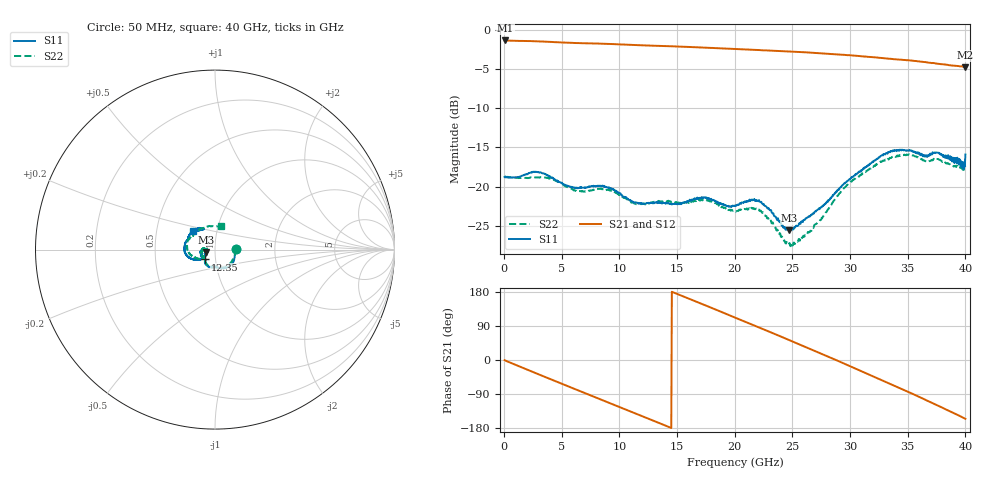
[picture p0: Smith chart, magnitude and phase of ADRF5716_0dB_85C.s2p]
! Device: ADRF5716
! Description: 30GHz 2-Bit Digital Attenuator
! Frequency: 100 MHz – 30 GHz
! Ports:
! ATTIN  = Port 1
! ATTOUT = Port 2
! State: 0 dB Attenuation selected
! Supply Voltage:
! VDD  =  +3.30 Volts
! VSS  =  -3.30 Volts
! Control Voltages:
! D5 = 0V, D6 = 0V
! Temperature = +85 C
! Data: Data was collected using a calibrated network analyzer.
!  The reference plane is the package pins of ADRF5716 switch.
! Note: Analog Devices supplies this data as a sample of measured data for this product.
!  Your particular data for this product may vary.
!  Analog Devices reserves the right to change this data at anytime
# HZ S DB R 50
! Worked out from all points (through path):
!   800 points, 50 MHz to 40 GHz, reference 50 ohm
!   highest |S21| = -1.40 dB at 100 MHz (marker M1); lowest = -4.8 dB at 40 GHz (marker M2)
!   group delay of S21, straight-line fit = 35.3 ps
!   lowest |S11| = -25.6 dB at 24.7 GHz (marker M3), VSWR 1.11, Z = 45.1 - j1.13 ohm
!   |S11| at or under -10 dB: start of sweep to end of sweep
!   |S22| runs from -27.6 to -15.9 dB; largest |S21 - S12| = 0
!   S11 on the Smith chart (normalised r, x): 50 MHz: 1.26, +0.01; 12.35 GHz: 0.89, -0.10; 40 GHz: 0.77, +0.16
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5e7  -18.79 1.2  -1.40 -0.6  -1.40 -0.6  -18.74 1.9
1e8  -18.76 -1.4  -1.40 -1.4  -1.40 -1.4  -18.73 -1.5
1.9e9  -18.45 -26.0  -1.46 -24.0  -1.46 -24.0  -18.89 -28.0
3.75e9  -18.53 -59.8  -1.56 -47.2  -1.56 -47.2  -18.92 -56.3
6.75e9  -20.13 -91.8  -1.74 -84.1  -1.74 -84.1  -20.65 -91.0
9.35e9  -20.31 -120.7  -1.85 -116.0  -1.85 -116.0  -20.55 -118.8
1.235e10  -22.12 -135.5  -2.03 -152.8  -2.03 -152.8  -22.13 -135.5
1.34e10  -22.05 -140.3  -2.08 -165.8  -2.08 -165.8  -21.83 -141.7
1.49e10  -22.23 -145.6  -2.16 175.7  -2.16 175.7  -21.98 -150.6
1.655e10  -21.57 -150.6  -2.25 155.4  -2.25 155.4  -21.84 -157.2
1.84e10  -21.87 -162.4  -2.37 132.5  -2.37 132.5  -22.13 -170.6
2.005e10  -22.39 -161.9  -2.48 111.6  -2.48 111.6  -23.08 -172.9
2.225e10  -22.01 -174.0  -2.64 84.0  -2.64 84.0  -23.06 176.6
2.47e10  -25.56 -166.3  -2.81 52.8  -2.81 52.8  -27.31 -173.8
2.67e10  -23.59 -150.1  -2.97 27.0  -2.97 27.0  -25.47 -149.2
2.83e10  -21.46 -145.0  -3.12 6.2  -3.12 6.2  -22.56 -143.9
2.99e10  -19.14 -148.4  -3.27 -14.9  -3.27 -14.9  -19.57 -150.9
3.335e10  -15.64 -172.0  -3.72 -61.2  -3.72 -61.2  -16.56 -177.4
3.495e10  -15.38 170.7  -3.91 -82.7  -3.91 -82.7  -15.95 165.0
3.645e10  -16.03 158.4  -4.15 -103.7  -4.15 -103.7  -16.69 148.8
3.84e10  -16.14 137.3  -4.49 -131.8  -4.49 -131.8  -17.08 126.1
4e10  -15.91 140.4  -4.79 -155.1  -4.79 -155.1  -17.45 75.7
